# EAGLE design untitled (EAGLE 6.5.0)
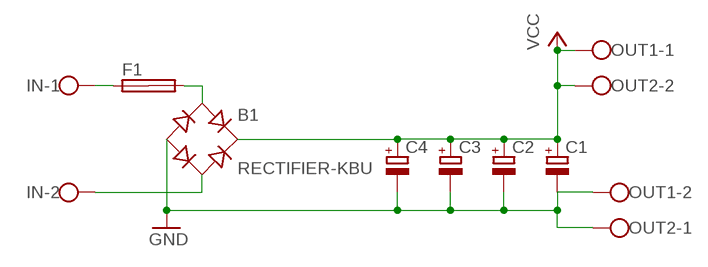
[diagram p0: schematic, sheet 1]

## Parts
B1  RECTIFIER-KBU  [KBU]
C1  CPOL-EUE7.5-18  [E7,5-18]
C2  CPOL-EUE7.5-18  [E7,5-18]
C3  CPOL-EUE7.5-18  [E7,5-18]
C4  CPOL-EUE7.5-18  [E7,5-18]
F1  SHK20L  [SHK20L]
IN  W237-102  [W237-102]
OUT1  W237-102  [W237-102]
OUT2  W237-102  [W237-102]

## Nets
GND: B1.- C1.- C2.- C3.- C4.- OUT1.2 OUT2.1
N$1: B1.AC1 F1.2A
N$2: B1.AC2 IN.2
N$4: F1.1A IN.1
VCC: B1.+ C1.+ C2.+ C3.+ C4.+ OUT1.1 OUT2.2
Unconnected: F1.1B F1.2B

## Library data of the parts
B1 = rectifier:RECTIFIER-: Rectifier
C1-C4 = resistor:CPOL-EU: POLARIZED CAPACITOR, European symbol
F1 = fuse:SHK20L: FUSE HOLDER 5 x 20 mm, SH contact, SHH1 Schukat, E1073 Buerklin; OC_FARNELL: unknown; OC_NEWARK: unknown
IN OUT1 OUT2 = con-wago-500:W237-102: WAGO SCREW CLAMP; MPN: 237-102; OC_FARNELL: unknown; OC_NEWARK: 70K9898

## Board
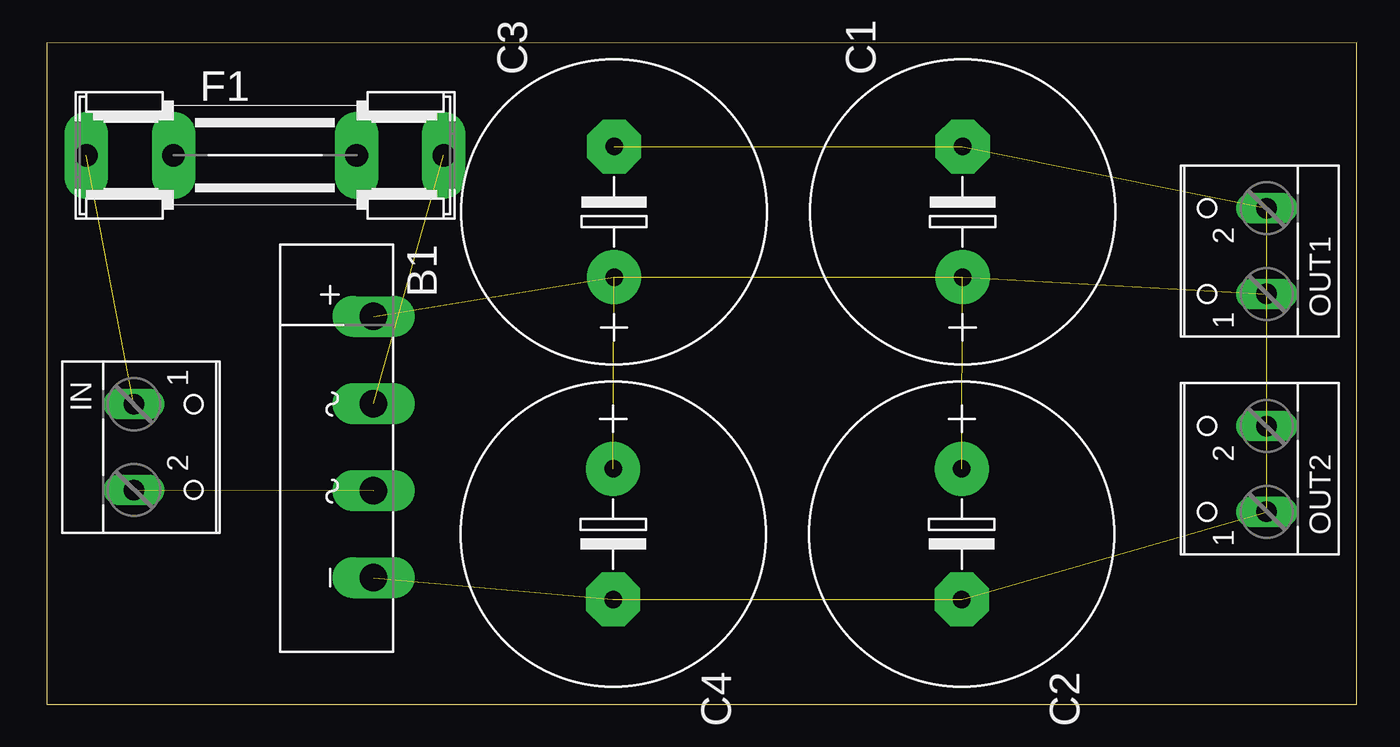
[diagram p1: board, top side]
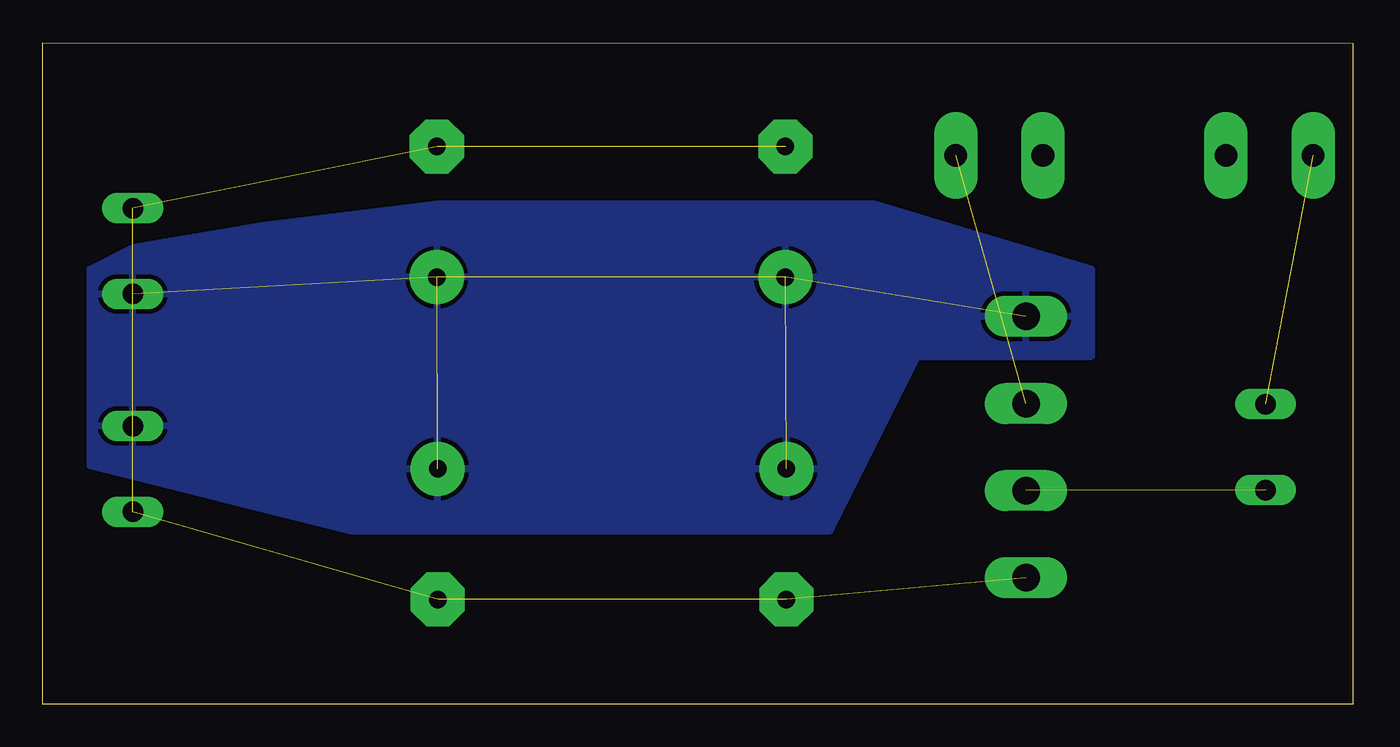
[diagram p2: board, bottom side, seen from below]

Size 76.36 x 38.56 mm. Coordinates in mm from the lower left corner, seen from the top.
Outline: 0,0 76.36,0 76.36,38.56 0,38.53 0,0
Copper layers (1*16): Top 0.035mm / dielectric 1.5mm / Bottom 0.035mm
Design rules "default": minimum track width 10mil, minimum drill 24mil, track to track 8mil, track to pad 8mil, pad to pad 8mil, via to via 8mil, smd to smd 8mil, copper to edge 40mil, drill to drill 8mil, minimum pad ring 10mil, minimum via ring 8mil, stop-mask expansion 4mil, vias tented up to drill 0mil, thermal gap 10mil

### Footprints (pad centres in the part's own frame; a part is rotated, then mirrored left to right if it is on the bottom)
KBU = drill 1.6 long: + -7.62,2.54; - 7.62,2.54; AC1 -2.54,2.54; AC2 2.54,2.54
E7,5-18 = drill 1.016 pad 3.15: + -3.81,0 | drill 1.016 pad 3.15 octagon: - 3.81,0
SHK20L = drill 1.321 pad 2.54 long: 1A -10.414,0; 1B -5.334,0; 2A 10.414,0; 2B 5.334,0
W237-102 = drill 1.194 long: 1 -2.5,-1.27; 2 2.5,-1.27

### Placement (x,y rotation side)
B1  16.51,14.99 270 top
C1  53.39,28.7 90 top
C2  53.34,9.91 270 top
C3  33.07,28.7 90 top
C4  33.02,9.91 270 top
F1  12.73,32 0 top
IN  6.35,14.99 270 top
OUT1  69.85,26.42 90 top
OUT2  69.85,13.72 90 top

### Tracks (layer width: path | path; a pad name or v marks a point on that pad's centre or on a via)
GND  (6 unrouted)
N$1  (1 unrouted)
N$2  (1 unrouted)
N$4  (1 unrouted)
VCC  (6 unrouted)
  pour Bottom: 27.91,29.16 53.31,29.16 63.47,27.89 71.09,26.62 73.63,25.35 73.63,13.92 58.39,10.11 30.45,10.11 25.37,20.27 15.21,20.27 15.21,25.35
